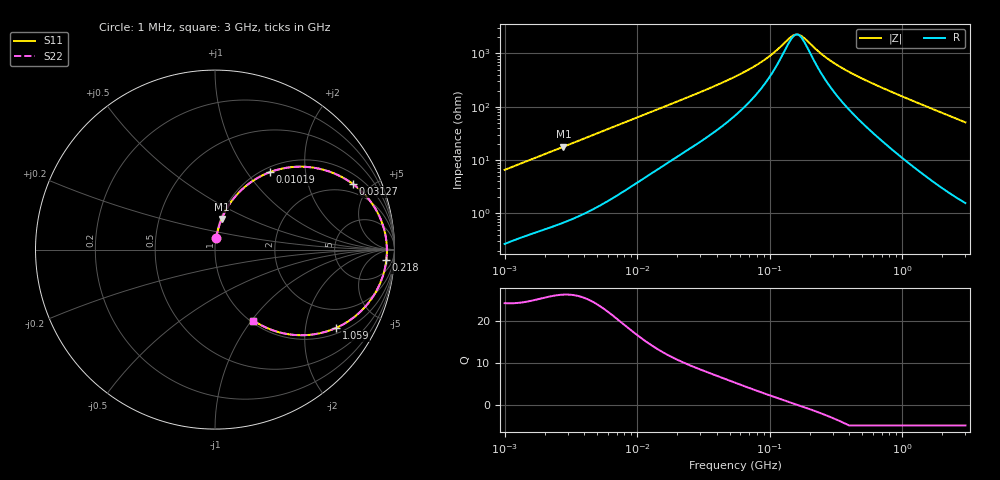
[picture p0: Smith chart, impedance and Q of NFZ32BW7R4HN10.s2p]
! NFZ32BW7R4HN10
# Hz S RI R 50
!Freq.(Hz) S11(Real) S11(Imag) S21(Real) S21(Imag) S12(Real) S12(Imag) S22(Real) S22(Imag)
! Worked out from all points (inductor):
!   401 points, 1 MHz to 3 GHz, reference 50 ohm
!   read as one part in series: L = 1.04 uH near 1.041 MHz
!   highest Q = 26.5 at 2.775 MHz (marker M1), where L = 1.02 uH
!   self-resonance near 160.3 MHz
!   S11 on the Smith chart (normalised r, x): 1 MHz: 1.01, +0.13; 10.19 MHz: 1.08, +1.29; 31.27 MHz: 1.47, +3.91; 218 MHz: 15, -21; 1.059 GHz: 1.20, -2.94; 3 GHz: 1.03, -1.02
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1000000  0.00693 0.065  0.9931 -0.065  0.9931 -0.065  0.00693 0.065
2775447  0.0367 0.1701  0.9633 -0.1701  0.9633 -0.1701  0.0367 0.1701
3823119  0.064 0.2262  0.936 -0.2262  0.936 -0.2262  0.064 0.2262
6305767  0.1494 0.3343  0.8506 -0.3343  0.8506 -0.3343  0.1494 0.3343
1.019448e7  0.3039 0.4307  0.6961 -0.4307  0.6961 -0.4307  0.3039 0.4307
1.461624e7  0.4605 0.4619  0.5395 -0.4619  0.5395 -0.4619  0.4605 0.4619
2.054061e7  0.6127 0.4425  0.3873 -0.4425  0.3873 -0.4425  0.6127 0.4425
3.127247e7  0.7685 0.3654  0.2315 -0.3654  0.2315 -0.3654  0.7685 0.3654
5.477226e7  0.8935 0.228  0.1065 -0.228  0.1065 -0.228  0.8935 0.228
7.248696e7  0.9261 0.162  0.0739 -0.162  0.0739 -0.162  0.9261 0.162
9.216659e7  0.9433 0.1096  0.0567 -0.1096  0.0567 -0.1096  0.9433 0.1096
1.520175e8  0.9576 0.0102  0.0424 -0.0102  0.0424 -0.0102  0.9576 0.0102
1.714156e8  0.9577 -0.0129  0.0423 0.0129  0.0423 0.0129  0.9577 -0.0129
2.094008e8  0.9553 -0.0518  0.0447 0.0518  0.0447 0.0518  0.9553 -0.0518
2.179536e8  0.9544 -0.0598  0.0456 0.0598  0.0456 0.0598  0.9544 -0.0598
2.771263e8  0.9457 -0.1092  0.0543 0.1092  0.0543 0.1092  0.9457 -0.1092
3.667557e8  0.9264 -0.1721  0.0736 0.1721  0.0736 0.1721  0.9264 -0.1721
5.583748e8  0.8687 -0.2787  0.1313 0.2787  0.1313 0.2787  0.8687 -0.2787
8.005644e8  0.7777 -0.3741  0.2223 0.3741  0.2223 0.3741  0.7777 -0.3741
1.059487e9  0.6742 -0.4365  0.3258 0.4365  0.3258 0.4365  0.6742 -0.4365
1.712864e9  0.4498 -0.4761  0.5502 0.4761  0.5502 0.4761  0.4498 -0.4761
3e9  0.2143 -0.3953  0.7857 0.3953  0.7857 0.3953  0.2143 -0.3953
